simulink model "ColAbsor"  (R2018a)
settings: Solver=VariableStepAuto  StartTime=0.0  StopTime=10  RelTol=1e-3
undefined symbols (not defined in the file): a824, af47, c3559468a7ef, ColAbsor, d552541c, sdiscope

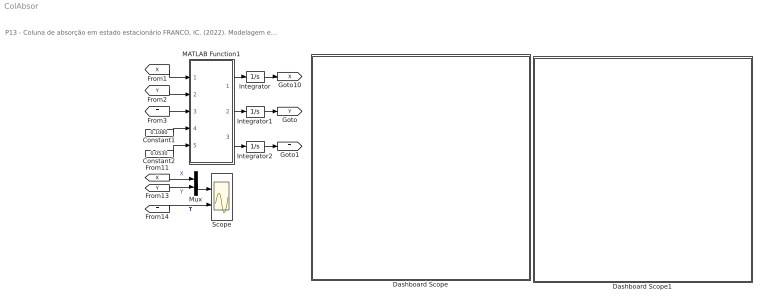
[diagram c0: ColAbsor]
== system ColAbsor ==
  note: P13 - Coluna de absorção em estado estacionário FRANCO, IC. (2022). Modelagem e Simulação: Problemas Típicos da Engenharia Química para Simulação e Análise. NOTAS DE AULA INOVADORAS. The Journal of Engineering and Exact Sciences. Material Complementar.
  Constant1 : Constant  Value=0.1080
  Constant2 : Constant  Value=0.0530
  Dashboard Scope : Subsystem  DialogController=hmiCreateDDGDialog  IsWebBlock=on  mask(MWDashboardBlock){webBlockId=d552541c-0130-4049-87af-c3559468a7ef, webBlockType=sdiscope, ShowInitialText=on, HMISrcModelName=ColAbsor}
      mask prompts: webBlockId "WebBlock Id"; webBlockType "WebBlock Type"; HMISrcModelName "Source Model"
      mask help: SimulinkHMI:dialogs:HMIScopeDialogDesc
  Dashboard Scope1 : Subsystem  DialogController=hmiCreateDDGDialog  IsWebBlock=on  mask(MWDashboardBlock){webBlockId=0b3540ed-a824-4f2a-af47-2b9e6c7fcd95, webBlockType=sdiscope, ShowInitialText=on, HMISrcModelName=ColAbsor}
      mask prompts: webBlockId "WebBlock Id"; webBlockType "WebBlock Type"; HMISrcModelName "Source Model"
      mask help: SimulinkHMI:dialogs:HMIScopeDialogDesc
  Integrator : Integrator
  Integrator1 : Integrator  InitialCondition=0.00263
  Integrator2 : Integrator  InitialCondition=20
  MATLAB Function1 : MATLAB Function  TreatAsAtomicUnit=on
  Mux : Mux  Inputs=2
  Scope : Scope  NumInputPorts=2
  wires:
  MATLAB Function1/1(dX) -> Integrator/1
  Integrator/1 -> [X]
  [X] -> MATLAB Function1/1(X)
  MATLAB Function1/2(dY) -> Integrator1/1
  Integrator1/1 -> [Y]
  [Y] -> MATLAB Function1/2(Y)
  [T] -> MATLAB Function1/3(T)
  MATLAB Function1/3(dT) -> Integrator2/1
  Integrator2/1 -> [T]
  Constant1/1 -> MATLAB Function1/4(Lm)
  [T] -> Scope/2  "T"
  [X] -> Mux/1  "X"
  [Y] -> Mux/2  "Y"
  Constant2/1 -> MATLAB Function1/5(Gm)
  Mux/1 -> Scope/1

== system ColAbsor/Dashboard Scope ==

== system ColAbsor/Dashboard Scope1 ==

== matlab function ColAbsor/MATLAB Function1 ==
function [dX,dY,dT]=fcn(X,Y,T,Lm,Gm)
%% Parâmetros
a     =     3.0100;
b     =    -0.1227;
c     =     0.0059;
Cp    =    75.2400;
KGa   =     0.1130;
PT    =   101.3300;
dHabs = 36200.0000;

%% equações auxiliares
% constante de equilíbrio
K=a+b*T+c*T^2;
% fração molar da fase líquida e da fase gasosa
x=X/(1+X);
y=Y/(1+Y);
% relação de equilíbrio
ye = K*x/PT;

%% Modelo matemático
dX = KGa*(y-ye)/Gm;
dY = KGa*(y-ye)/Lm;
dT = KGa*(y-ye)*dHabs/(Lm*Cp);
end
